FUNCTION_BLOCK FB_DO_IED_LD1_MMXU1_TotW EXTENDS FB_AcsiCommonDataClass
VAR_INPUT
	mag: FB_AcsiDATypeAnalogueValue := (fc:=ACSI_FC_MX, TrgOp:=ACSI_TrgOp_dchg OR ACSI_TrgOp_dupd, bLinkResult:=THIS^.AddDataToContainer(ipData:=mag));
	q: FB_AcsiDATypeQuality := (fc:=ACSI_FC_MX, TrgOp:=ACSI_TrgOp_qchg, bLinkResult:=THIS^.AddDataToContainer(ipData:=q));
	t: FB_AcsiDATypeTimeStamp := (fc:=ACSI_FC_MX, bLinkResult:=THIS^.AddDataToContainer(ipData:=t));
	units: FB_AcsiDATypeUnit := (fc:=ACSI_FC_CF, TrgOp:=ACSI_TrgOp_dchg, SIUnit:=(eValue:=E_AcsiSIUnit.Volt), multiplier:=(eValue:=E_AcsiMultiplier.Milli, bPresence:=TRUE), bLinkResult:=THIS^.AddDataToContainer(ipData:=units));
END_VAR
VAR
END_VAR

END_FUNCTION_BLOCK
